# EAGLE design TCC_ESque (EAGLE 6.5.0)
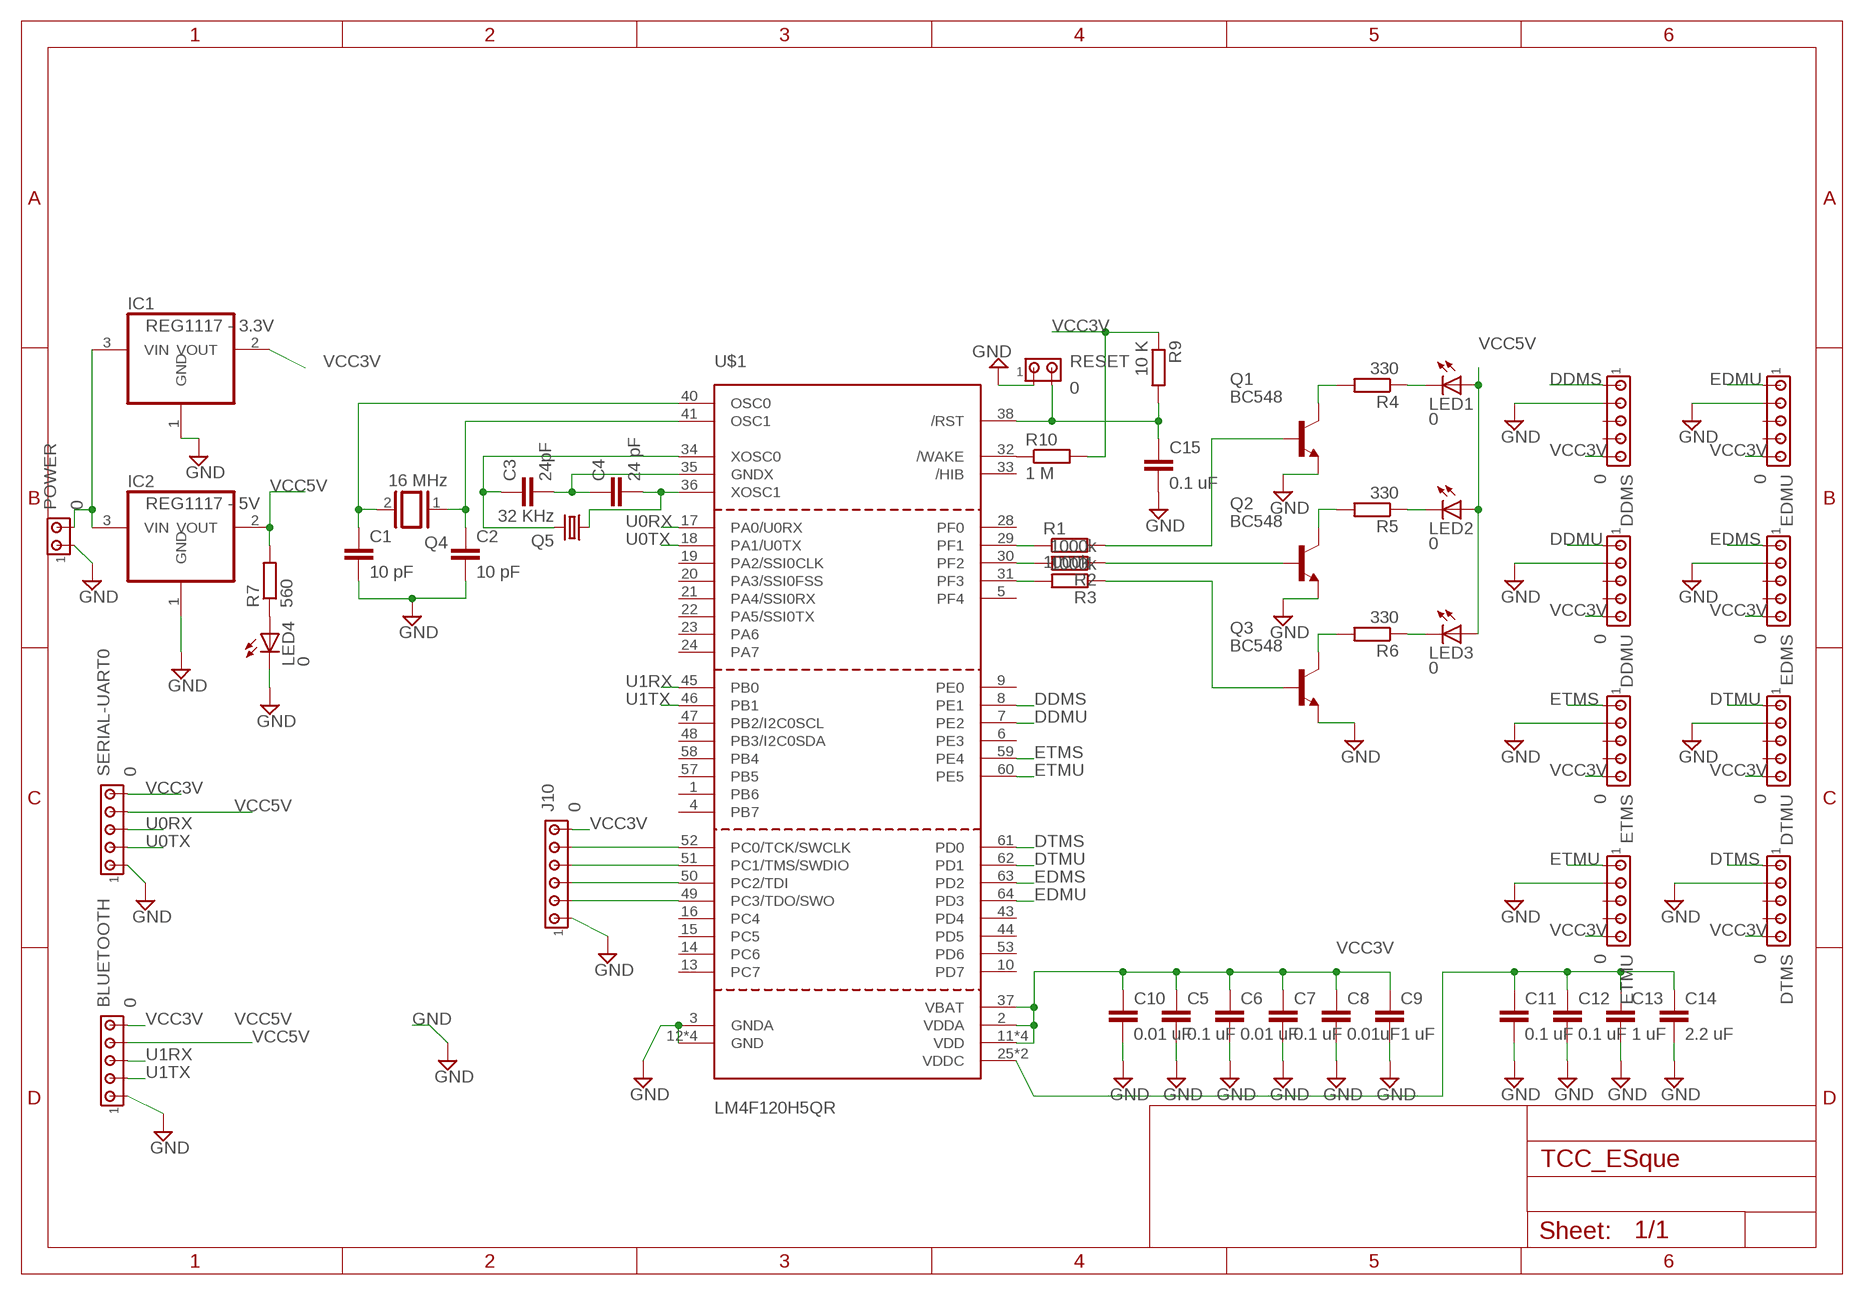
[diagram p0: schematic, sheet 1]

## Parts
BLUETOOTH  0  MTA05-100  [10X05MTA]
C1  10 pF  C2.5/6  [C2.5-6]
C2  10 pF  C2.5/6  [C2.5-6]
C3  24pF  C2.5/6  [C2.5-6]
C4  24 pF  C2.5/6  [C2.5-6]
C5  0.1 uF  C2.5/6  [C2.5-6]
C6  0.01 uF  C2.5/6  [C2.5-6]
C7  0.1 uF  C2.5/6  [C2.5-6]
C8  0.01uF  C2.5/6  [C2.5-6]
C9  1 uF  C2.5/6  [C2.5-6]
C10  0.01 uF  C2.5/6  [C2.5-6]
C11  0.1 uF  C2.5/6  [C2.5-6]
C12  0.1 uF  C2.5/6  [C2.5-6]
C13  1 uF  C2.5/6  [C2.5-6]
C14  2.2 uF  C2.5/6  [C2.5-6]
C15  0.1 uF  C2.5/6  [C2.5-6]
DDMS  0  MTA05-100  [10X05MTA]
DDMU  0  MTA05-100  [10X05MTA]
DTMS  0  MTA05-100  [10X05MTA]
DTMU  0  MTA05-100  [10X05MTA]
EDMS  0  MTA05-100  [10X05MTA]
EDMU  0  MTA05-100  [10X05MTA]
ETMS  0  MTA05-100  [10X05MTA]
ETMU  0  MTA05-100  [10X05MTA]
IC1  REG1117 - 3.3V  REG1117  [SOT223]
IC2  REG1117 - 5V  REG1117  [SOT223]
J10  0  MTA06-100  [10X06MTA]
LED1  0  LED5MM  [LED5MM]
LED2  0  LED5MM  [LED5MM]
LED3  0  LED5MM  [LED5MM]
LED4  0  LED5MM  [LED5MM]
POWER  0  MTA02-156  [1X2MTA]
Q1  BC548  [TO92-EBC]
Q2  BC548  [TO92-EBC]
Q3  BC548  [TO92-EBC]
Q4  16 MHz  XTAL/S  [QS]
Q5  32 KHz  CRYSTALTC26H  [TC26H]
R1  1000k  R-EU_0204/7  [0204/7]
R2  1000k  R-EU_0204/7  [0204/7]
R3  1000k  R-EU_0204/7  [0204/7]
R4  330  R-EU_0204/7  [0204/7]
R5  330  R-EU_0204/7  [0204/7]
R6  330  R-EU_0204/7  [0204/7]
R7  560  R-EU_0204/7  [0204/7]
R9  10 K  R-EU_0204/7  [0204/7]
R10  1 M  R-EU_0204/7  [0204/7]
RESET  0  MTA02-156  [1X2MTA]
SERIAL-UART0  0  MTA05-100  [10X05MTA]
U$1  LM4F120H5QR  [LQFP64]

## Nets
DDMS: DDMS.1 U$1.8(PE1)
DDMU: DDMU.1 U$1.7(PE2)
DTMS: DTMS.1 U$1.61(PD0)
DTMU: DTMU.1 U$1.62(PD1)
EDMS: EDMS.1 U$1.63(PD2)
EDMU: EDMU.1 U$1.64(PD3)
ETMS: ETMS.1 U$1.59(PE4)
ETMU: ETMU.1 U$1.60(PE5)
GND: BLUETOOTH.1 C1.2 C2.2 C5.2 C6.2 C7.2 C8.2 C9.2 C10.2 C11.2 C12.2 C13.2 C14.2 C15.2 DDMS.2 DDMU.2 DTMS.2 DTMU.2 EDMS.2 EDMU.2 ETMS.2 ETMU.2 IC1.1(GND) IC2.1(GND) J10.6 LED4.K(C) POWER.1 Q1.E Q2.E Q3.E RESET.1 SERIAL-UART0.1 U$1.3(GNDA) U$1.12(GND) U$1.27(GND) U$1.39(GND) U$1.55(GND)
JTAG: J10.2 U$1.52(PC0/TCK/SWCLK)
N$1: R1.1 U$1.29(PF1)
N$2: R2.2 U$1.30(PF2)
N$3: R3.2 U$1.31(PF3)
N$4: Q1.B R1.2
N$5: C1.1 Q4.2 U$1.40(OSC0)
N$6: J10.5 U$1.49(PC3/TDO/SWO)
N$7: C3.1 Q5.2 U$1.34(XOSC0)
N$8: C4.2 Q5.1 U$1.36(XOSC1)
N$9: Q2.B R2.1
N$10: Q3.B R3.1
N$11: C3.2 C4.1 U$1.35(GNDX)
N$12: Q1.C R4.2
N$13: LED1.K(C) R4.1
N$14: LED4.A R7.1
N$15: J10.4 U$1.50(PC2/TDI)
N$16: Q2.C R5.2
N$17: Q3.C R6.2
N$18: LED3.K(C) R6.1
N$19: LED2.K(C) R5.1
N$20: J10.3 U$1.51(PC1/TMS/SWDIO)
N$21: R10.1 U$1.32(/WAKE)
N$22: C15.1 R9.2 RESET.2 U$1.38(/RST)
N$23: IC1.3(VIN) IC2.3(VIN) POWER.2
N$24: C11.1 C12.1 C13.1 C14.1 U$1.25(VDDC) U$1.56(VDDC)
N$25: C2.1 Q4.1 U$1.41(OSC1)
U0RX: SERIAL-UART0.3 U$1.17(PA0/U0RX)
U0TX: SERIAL-UART0.2 U$1.18(PA1/U0TX)
U1RX: BLUETOOTH.3 U$1.45(PB0)
U1TX: BLUETOOTH.2 U$1.46(PB1)
VCC3V: BLUETOOTH.5 C5.1 C6.1 C7.1 C8.1 C9.1 C10.1 DDMS.5 DDMU.5 DTMS.5 DTMU.5 EDMS.5 EDMU.5 ETMS.5 ETMU.5 IC1.2(VOUT) J10.1 R9.1 R10.2 SERIAL-UART0.5 U$1.2(VDDA) U$1.11(VDD) U$1.26(VDD) U$1.37(VBAT) U$1.42(VDD) U$1.54(VDD)
VCC5V: BLUETOOTH.4 IC2.2(VOUT) LED1.A LED2.A LED3.A R7.2 SERIAL-UART0.4
Unconnected: DDMS.3 DDMS.4 DDMU.3 DDMU.4 DTMS.3 DTMS.4 DTMU.3 DTMU.4 EDMS.3 EDMS.4 EDMU.3 EDMU.4 ETMS.3 ETMS.4 ETMU.3 ETMU.4 U$1.1(PB6) U$1.4(PB7) U$1.5(PF4) U$1.6(PE3) U$1.9(PE0) U$1.10(PD7) U$1.13(PC7) U$1.14(PC6) U$1.15(PC5) U$1.16(PC4) U$1.19(PA2/SSI0CLK) U$1.20(PA3/SSI0FSS) U$1.21(PA4/SSI0RX) U$1.22(PA5/SSI0TX) U$1.23(PA6) U$1.24(PA7) U$1.28(PF0) U$1.33(/HIB) U$1.43(PD4) U$1.44(PD5) U$1.47(PB2/I2C0SCL) U$1.48(PB3/I2C0SDA) U$1.53(PD6) U$1.57(PB5) U$1.58(PB4)

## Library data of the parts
BLUETOOTH DDMS DDMU DTMS DTMU EDMS EDMU ETMS ETMU SERIAL-UART0 = con-amp:MTA05-100: AMP connector
C1-C15 = capacitor-wima:C: CAPACITOR
IC1 IC2 = burr-brown:REG1117: 800mA and 1A Low Dropout (LDO) Positive Regulator 1.8V, 2.5V, 2.85V, 3.3V, 5V, and Adj; MPN: REG1117; OC_FARNELL: 1097566; OC_NEWARK: 14P6981
J10 = con-amp:MTA06-100: AMP connector
LED1-LED4 = led:LED: LED
POWER RESET = con-amp:MTA02-156: AMP connector
Q1-Q3 = transistor-npn:BC548*: NPN Transistor
Q4 = special:XTAL/S: CRYSTAL
Q5 = crystal:CRYSTAL: CRYSTAL; OC_FARNELL: unknown; OC_NEWARK: unknown
R1 = resistor:R-EU_: RESISTOR, European symbol
R2-R7 R9 R10 = rcl:R-EU_: RESISTOR, European symbol
U$1 = fabhack:LM4F120H5QR: LM4F120H5QR Cortex-M4F from the LM4F120 Series.

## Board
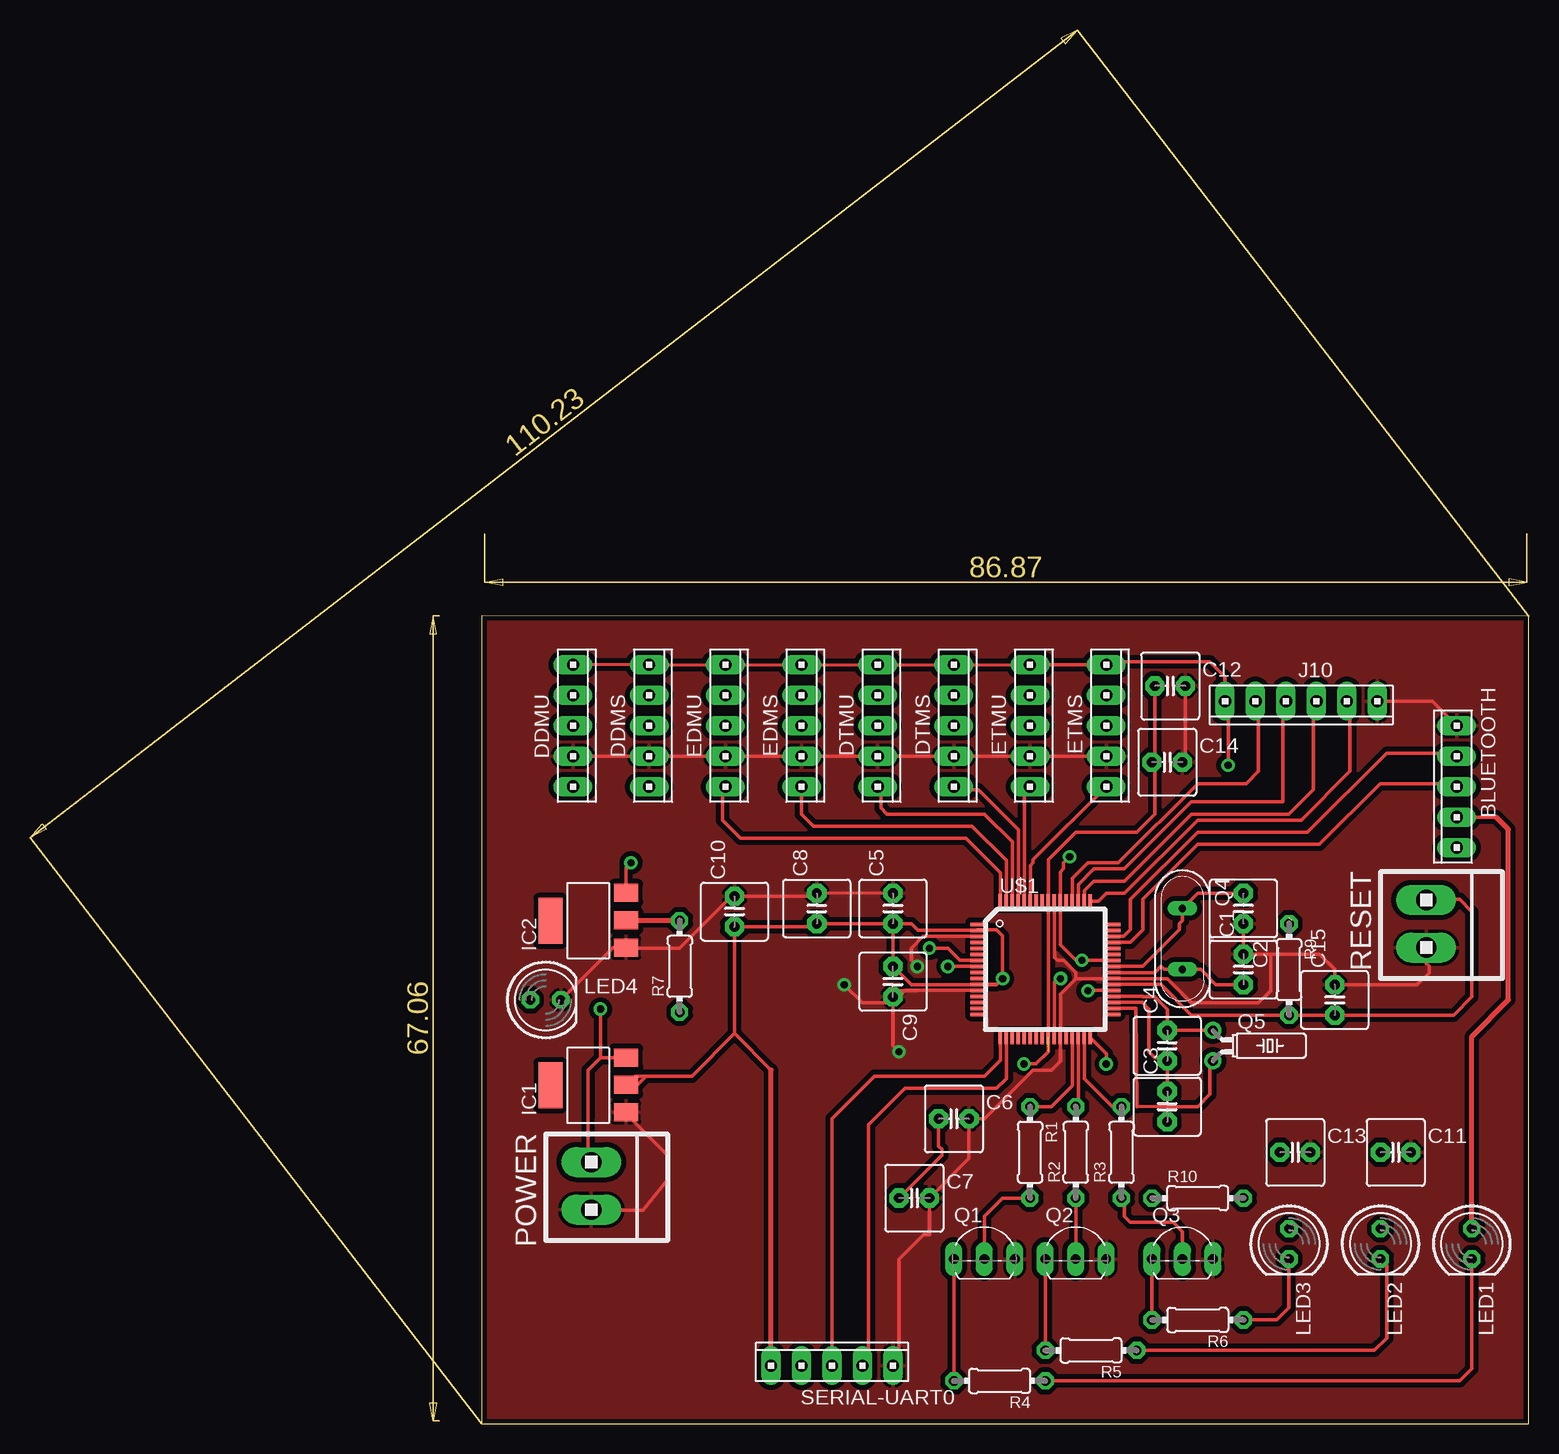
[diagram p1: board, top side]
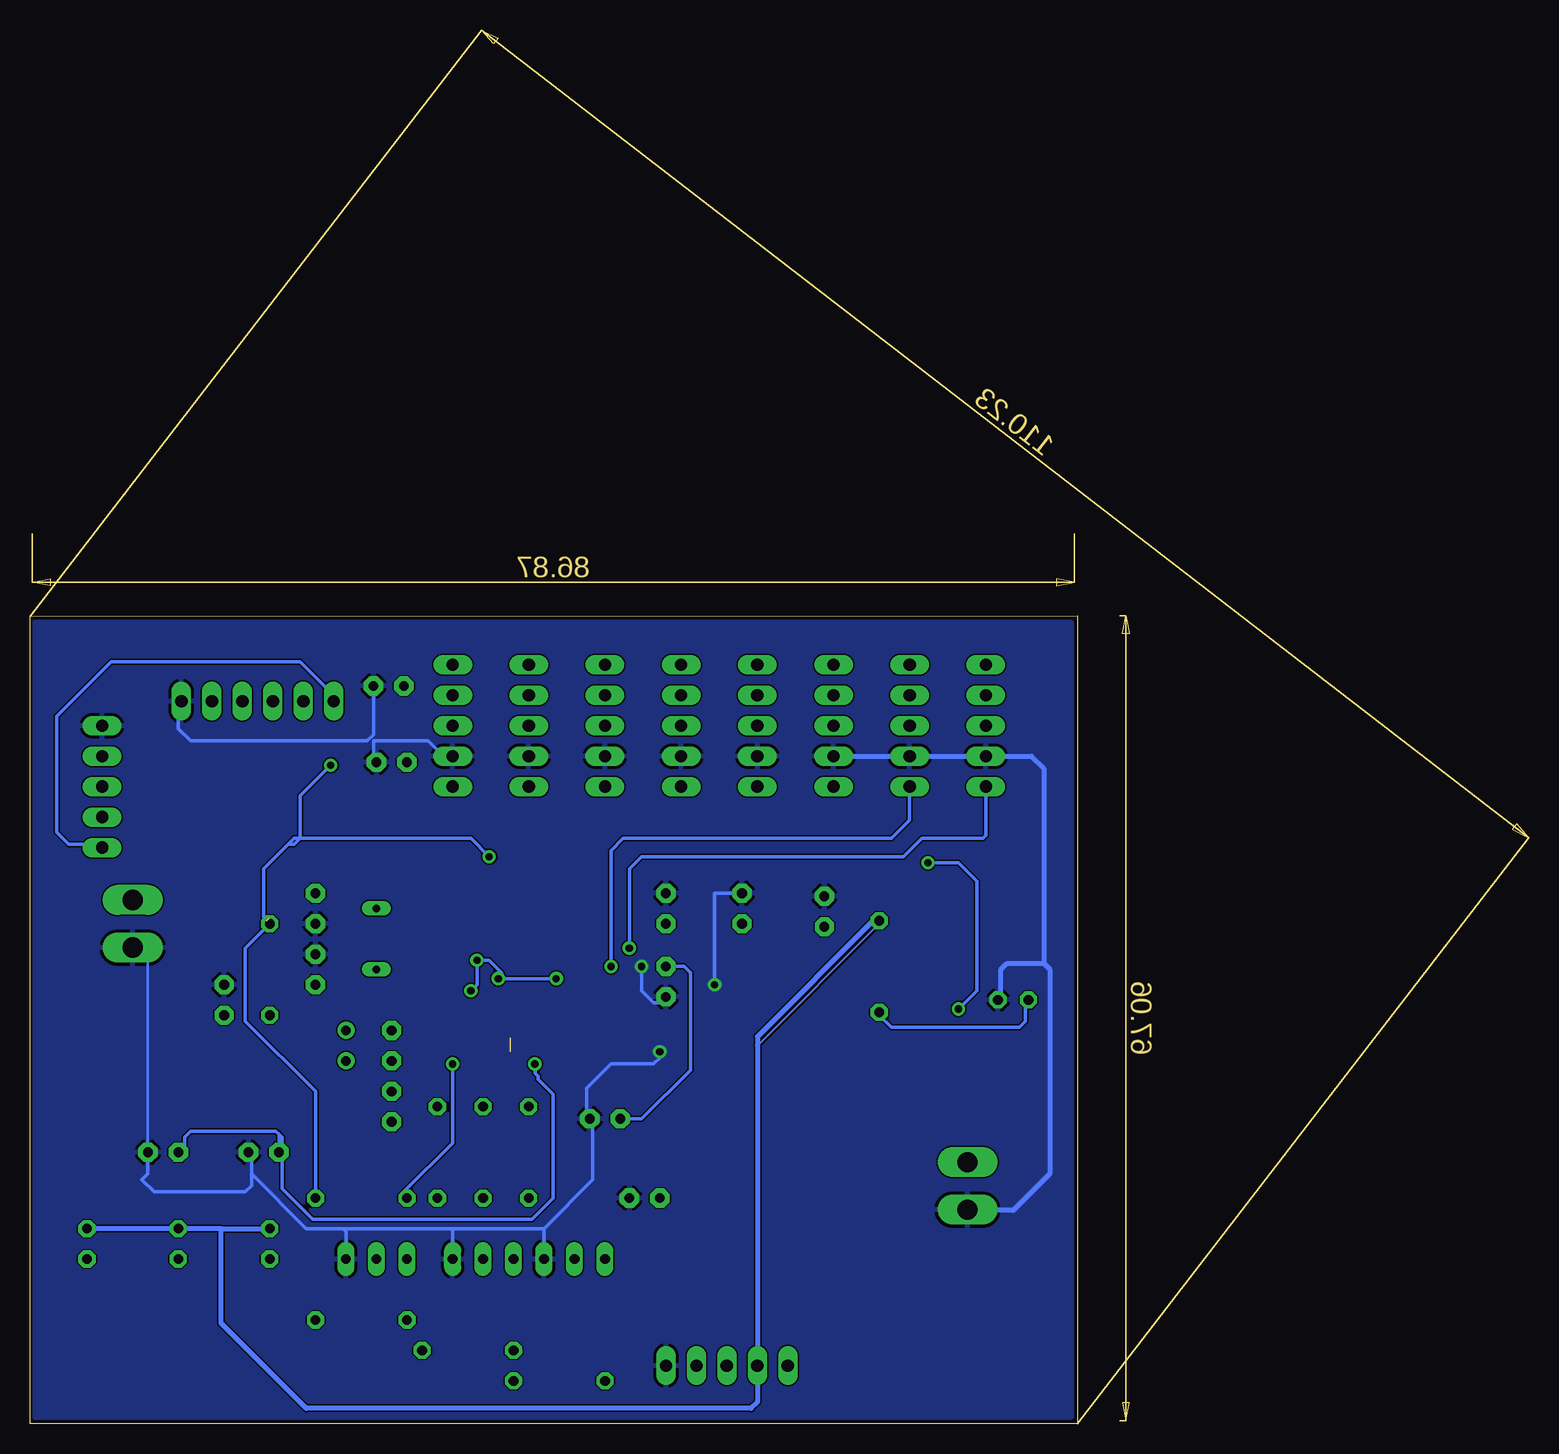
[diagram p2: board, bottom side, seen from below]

Size 124.95 x 116.13 mm. Coordinates in mm from the lower left corner, seen from the top.
Outline: 37.65,0 124.95,0 124.95,67.3 37.64,67.31 37.65,0
Copper layers (1*16): Top 0.035mm / dielectric 1.5mm / Bottom 0.035mm
Design rules "SparkFun *": minimum track width 8mil, minimum drill 23mil, track to track 5mil, track to pad 5mil, pad to pad 5mil, via to via 5mil, smd to smd 5mil, copper to edge 5mil, drill to drill 5mil, minimum pad ring 12mil, minimum via ring 10mil, stop-mask expansion 4mil, vias tented up to drill 20mil, thermal gap 10mil

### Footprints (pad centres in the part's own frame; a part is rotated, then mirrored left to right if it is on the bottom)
10X05MTA = drill 1.016 long: 1 5.08,0; 2 2.54,0; 3 0,0; 4 -2.54,0; 5 -5.08,0
C2.5-6 = drill 0.813 pad 1.6 octagon: 1 -1.27,0; 2 1.27,0
SOT223 = smd 1.499 x 2.007: 1 -2.261,-3.15; 2 0.025,-3.15; 3 2.311,-3.15 | smd 3.81 x 2.007: 4 0,3.15
10X06MTA = drill 1.016 long: 1 6.35,0; 2 3.81,0; 3 1.27,0; 4 -1.27,0; 5 -3.81,0; 6 -6.35,0
LED5MM = drill 0.813 octagon: A -1.27,0; K 1.27,0
1X2MTA = drill 1.676 long: 1 1.981,0; 2 -1.981,0
TO92-EBC = drill 0.813 long: B 0,-1.27; C -2.54,-1.27; E 2.54,-1.27
QS = drill 0.61 long: 1 -2.54,0; 2 2.54,0
TC26H = drill 0.813: 1 -1.27,0; 2 1.27,0
0204/7 = drill 0.813 octagon: 1 -3.81,0; 2 3.81,0
LQFP64 = smd 1.1 x 0.285: 1 -5.7,3.75; 2 -5.7,3.25; 3 -5.7,2.75; 4 -5.7,2.25; 5 -5.7,1.75; 6 -5.7,1.25; 7 -5.7,0.75; 8 -5.7,0.25; 9 -5.7,-0.25; 10 -5.7,-0.75; 11 -5.7,-1.25; 12 -5.7,-1.75; 13 -5.7,-2.25; 14 -5.7,-2.75; 15 -5.7,-3.25; 16 -5.7,-3.75; 33 5.7,-3.75; 34 5.7,-3.25; 35 5.7,-2.75; 36 5.7,-2.25; 37 5.7,-1.75; 38 5.7,-1.25; 39 5.7,-0.75; 40 5.7,-0.25; 41 5.7,0.25; 42 5.7,0.75; 43 5.7,1.25; 44 5.7,1.75; 45 5.7,2.25; 46 5.7,2.75; 47 5.7,3.25; 48 5.7,3.75 | smd 0.285 x 1.1: 17 -3.75,-5.7; 18 -3.25,-5.7; 19 -2.75,-5.7; 20 -2.25,-5.7; 21 -1.75,-5.7; 22 -1.25,-5.7; 23 -0.75,-5.7; 24 -0.25,-5.7; 25 0.25,-5.7; 26 0.75,-5.7; 27 1.25,-5.7; 28 1.75,-5.7; 29 2.25,-5.7; 30 2.75,-5.7; 31 3.25,-5.7; 32 3.75,-5.7; 49 3.75,5.7; 50 3.25,5.7; 51 2.75,5.7; 52 2.25,5.7; 53 1.75,5.7; 54 1.25,5.7; 55 0.75,5.7; 56 0.25,5.7; 57 -0.25,5.7; 58 -0.75,5.7; 59 -1.25,5.7; 60 -1.75,5.7; 61 -2.25,5.7; 62 -2.75,5.7; 63 -3.25,5.7; 64 -3.75,5.7

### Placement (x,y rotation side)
BLUETOOTH  118.93,53.09 90 top
C1  101.15,37.85 90 top
C2  101.15,42.93 270 top
C3  94.8,26.42 90 top
C4  94.8,31.5 90 top
C5  71.94,42.93 90 top
C6  77.02,25.4 0 top
C7  73.71,18.8 0 top
C8  65.59,42.93 90 top
C9  71.94,36.83 270 top
C10  58.73,42.67 90 top
C11  113.85,22.61 0 top
C12  95.05,61.47 0 top
C13  105.46,22.61 0 top
C14  94.8,55.12 0 top
C15  108.77,35.31 90 top
DDMS  51.62,58.17 270 top
DDMU  45.27,58.17 270 top
DTMS  77.02,58.17 270 top
DTMU  70.67,58.17 270 top
EDMS  64.32,58.17 270 top
EDMU  57.97,58.17 270 top
ETMS  89.72,58.17 270 top
ETMU  83.37,58.17 270 top
IC1  46.54,28.19 90 top
IC2  46.54,41.91 90 top
J10  105.97,60.2 180 top
LED1  120.2,14.99 270 top
LED2  112.58,14.99 270 top
LED3  104.96,14.99 270 top
LED4  42.98,35.31 0 top
POWER  46.79,19.81 270 top
Q1  79.56,14.99 0 top
Q2  87.18,14.99 0 top
Q3  96.07,14.99 0 top
Q4  96.07,40.39 270 top
Q5  98.61,31.5 270 top
R1  83.37,22.61 270 top
R2  87.18,22.61 90 top
R3  90.99,22.61 90 top
R4  80.83,3.56 180 top
R5  88.45,6.1 180 top
R6  97.34,8.64 180 top
R7  54.16,38.1 90 top
R9  104.96,37.85 270 top
R10  97.34,18.8 0 top
RESET  116.39,41.66 270 top
SERIAL-UART0  66.86,4.83 0 top
U$1  84.64,37.85 0 top

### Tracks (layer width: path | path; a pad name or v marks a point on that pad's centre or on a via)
DDMS  (via drill 0.6)
  Top 0.305: U$1.8 v76.51,38.1
  Bottom 0.305: v76.51,38.1 76.51,47.75 75.49,48.77 53.14,48.77 51.62,50.29 DDMS.1
DDMU  (via drill 0.6)
  Top 0.305: v74.98,39.62 76.51,39.62 77.52,38.61 78.92,38.61 U$1.7
  Bottom 0.305: DDMU.1 45.27,49.02 45.52,48.77 50.6,48.77 52.12,47.24 73.97,47.24 74.98,46.23 v74.98,39.62
DTMS
  Top 0.305: U$1.61 82.39,49.49 79.05,52.83 77.27,52.83 DTMS.1
DTMU
  Top 0.305: U$1.62 81.89,48.47 79.56,50.8 71.43,50.8 70.92,51.31 70.92,52.83 DTMU.1
EDMS
  Top 0.305: U$1.63 81.39,46.94 78.54,49.78 65.33,49.78 64.32,50.8 EDMS.1
EDMU
  Top 0.305: U$1.64 80.89,45.91 78.03,48.77 59.24,48.77 57.71,50.29 57.71,52.83 EDMU.1
ETMS
  Top 0.305: U$1.59 83.39,46.5 83.62,46.74 83.62,46.99 ETMS.1
ETMU
  Top 0.305: U$1.60 82.89,52.61 ETMU.1
GND  (via drill 0.6)
  Top 0.203: 50.35,25.15 50.35,26.42 IC1.1
  Top 0.254: C5.2 C8.2
  Top 0.305: C2.2 C1.2 103.43,39.12 | 103.43,39.12 107.5,39.12 108.77,37.85 C15.2 115.62,36.58 116.64,37.59 116.64,38.1 116.39,38.35 RESET.1 | 90.35,37.08 94.8,37.08 96.83,35.05 102.42,35.05 103.43,36.07 103.43,39.12 | 89.72,14.22 Q2.E | SERIAL-UART0.1 72.44,5.33 72.44,13.72 74.48,15.75 74.98,15.75 C7.2 78.29,22.1 C6.2 79.56,25.4 83.62,29.46 85.14,29.46 85.89,30.21 U$1.27 85.89,35.79 87.18,37.08 | 50.07,25.93 50.09,25.91 50.09,25.4 50.35,25.15 53.14,22.35 53.14,20.32 51.11,17.78 47.35,17.78 POWER.1 45.47,17.83 | C10.2 58.47,44.2 | LED4.K 48.59,39.65 IC2.1 49.71,39.62 54.16,39.62 58.47,43.94 C10.2 | C10.2 65.33,43.94 C8.2 | DDMU.2 DDMS.2 EDMU.2 EDMS.2 DTMU.2 DTMS.2 ETMU.2 ETMS.2 | C12.2 96.32,55.37 C14.2 | J10.6 116.89,60.2 BLUETOOTH.1 | v67.87,36.58 69.4,35.05 71.43,35.05 C9.2 72.44,36.07 73.97,36.07 74,36.1 U$1.12 72.98,36.1 71.94,35.05 71.94,31.5 v72.44,30.99 | U$1.3 74.43,40.6 73.46,39.62 73.46,38.61 v73.97,38.1 | U$1.55 85.39,38.87 85.65,38.61 86.16,38.61 87.18,37.59 87.18,37.08 | 87.18,37.08 90.32,37.08 U$1.39
  Bottom 0.203: C11.2 115.12,39.12 116.39,39.12 RESET.1
  Bottom 0.305: Q1.E 82.1,16.26 | 82.1,16.26 89.72,16.26 | 89.72,16.26 98.86,16.26 | 98.86,16.26 98.61,16 Q3.E | Q2.E 89.72,16.26 | 82.1,16.26 78.03,20.32 78.03,24.64 78.29,24.89 C6.2 78.54,25.65 78.54,27.94 76.51,29.97 72.95,29.97 72.44,30.48 v72.44,30.99 | ETMS.2 90.48,55.63 91.75,56.9 96.32,56.9 96.32,55.37 C14.2 | C12.2 96.32,57.4 96.83,56.9 111.56,56.9 112.58,57.91 112.58,59.94 J10.6 | 98.86,16.26 101.91,16.26 106.48,20.83 | 106.48,20.83 106.48,22.35 C13.2 | C11.2 115.12,20.83 115.62,20.32 114.61,19.3 106.99,19.3 106.48,19.81 106.48,20.83 | v67.87,36.58 67.87,44.2 C8.2 | v73.97,38.1 73.97,36.07 72.95,35.05 72.44,35.05 C9.2
  Bottom 0.406: LED4.K 44,35.31 44,37.85 43.49,38.35 40.44,38.35 | 40.44,38.35 39.93,37.85 39.93,20.83 42.98,17.78 46.74,17.78 POWER.1 | EDMU.2 41.46,55.63 40.44,54.61 40.44,38.35
  pour Top (isolate 0.406): 38.15,0.51 124.51,0.51 124.51,66.8 38.15,67.06
  pour Bottom: 38.41,66.8 38.15,66.8 38.15,0.51 124.51,0.51 124.51,66.8 38.15,66.8 38.15,66.55 38.41,66.8 38.15,66.8 38.15,66.29
JTAG
  Top 0.305: U$1.52 86.89,45.43 88.19,46.74 90.73,46.74 97.34,53.34 101.4,53.34 102.42,54.36 102.42,59.94 J10.2
N$1
  Top 0.305: U$1.29 86.89,28.16 85.14,26.42 R1.1
N$2
  Top 0.305: U$1.30 87.39,26.63 R2.2
N$3
  Top 0.305: U$1.31 87.89,28.75 90.22,26.42 R3.2
N$4
  Top 0.305: R1.2 81.08,18.8 79.56,17.27 Q1.B
N$5
  Top 0.305: C1.1 98.86,36.58 97.59,37.85 Q4.2 94.54,37.85 94.29,38.1 93.78,37.59 U$1.40
N$6
  Top 0.305: U$1.49 89.07,43.55 89.72,44.2 91.24,44.2 97.34,50.29 105.97,50.29 110.04,54.36 110.04,59.94 J10.5
N$7
  Top 0.254: C3.1 94.8,26.42 92.26,26.42 92.25,26.42
  Top 0.305: U$1.34 92.2,34.6 92.25,26.42 | 94.8,26.42 97.34,26.42 98.35,27.43 98.35,29.97 Q5.2
N$8
  Top 0.305: Q5.1 C4.2 94.8,34.54 93.78,35.56 92.76,35.56 92.73,35.6 U$1.36
N$9
  Top 0.305: R2.1 Q2.B
N$10
  Top 0.305: R3.1 91.24,18.54 91.24,17.27 91.75,16.76 95.3,16.76 96.07,16 Q3.B
N$11
  Top 0.305: C3.2 C4.1 94.54,30.48 93.78,30.48 93.27,30.99 93.27,34.54 92.72,35.1 U$1.35
N$12
  Top 0.305: Q1.C R4.2
N$13
  Top 0.305: R4.1 119.18,3.56 120.2,4.57 LED1.K
N$14
  Bottom 0.305: LED4.A 41.96,35.05 41.96,33.53 42.47,33.02 53.14,33.02 54.16,34.04 R7.1
N$15
  Top 0.305: U$1.50 87.89,44.4 88.7,45.21 91.24,45.21 96.83,50.8 104.96,50.8 106.99,52.83 106.99,59.94 J10.4
N$16
  Top 0.305: Q2.C R5.2
N$17
  Top 0.305: R6.2 Q3.C
N$18
  Top 0.305: R6.1 103.94,8.64 104.96,9.65 LED3.K
N$19
  Top 0.305: R5.1 112.07,6.1 113.08,7.11 113.08,13.21 LED2.K
N$20
  Top 0.305: U$1.51 87.39,44.91 88.7,46.23 91.24,46.23 96.83,51.82 104.45,51.82 104.45,59.94 J10.3
N$21  (via drill 0.6)
  Top 0.305: U$1.32 89.72,30.82 v89.72,29.97
  Bottom 0.305: v89.72,29.97 89.72,23.37 93.78,19.3 93.53,19.05 R10.1
N$22
  Top 0.305: U$1.38 94.27,36.6 96.83,34.04 R9.2 C15.1 118.67,34.04 120.2,35.56 120.2,42.67 119.18,43.69 116.44,43.69 RESET.2
N$23  (via drill 0.6)
  Top 0.305: POWER.2 46.54,22.05 46.54,29.46 47.55,30.48 | 47.55,30.48 47.58,30.51 IC1.3 49.66,30.48 47.55,30.48 | 47.55,30.48 v47.55,34.54 | v50.09,46.74 49.69,46.33 IC2.3
  Bottom 0.305: v47.55,34.54 46.03,36.07 46.03,45.21 47.55,46.74 v50.09,46.74
N$24  (via drill 0.6)  (1 unrouted)
  Top 0.305: C12.1 93.78,55.37 C14.1 93.78,54.86 93.78,50.8 92.26,49.28 87.18,49.28 84.89,46.99 U$1.56 84.89,30.99 83.87,29.97 v82.86,29.97
  Bottom 0.305: C13.1 104.19,24.13 | 104.19,24.13 104.45,24.38 111.56,24.38 112.07,23.88 112.07,23.11 C11.1 | 104.19,24.13 103.94,23.88 103.94,19.56 101.4,17.02 83.11,17.02 81.33,18.8 81.33,27.43 82.6,28.7 82.6,28.96 82.86,29.21 v82.86,29.97
N$25
  Top 0.305: U$1.41 92.76,38.1 95.81,41.15 95.81,41.66 96.07,41.91 Q4.1 97.34,44.2 C2.1
U0RX
  Top 0.305: SERIAL-UART0.3 66.86,25.4 70.41,28.96 79.56,28.96 80.89,30.29 U$1.17
U0TX
  Top 0.305: SERIAL-UART0.2 69.9,5.33 69.9,24.89 72.95,27.94 80.57,27.94 81.39,28.75 U$1.18
U1RX
  Top 0.305: U$1.45 91.71,40.1 92.76,41.15 92.76,43.69 97.34,48.26 107.5,48.26 112.58,53.34 118.67,53.34 BLUETOOTH.3
U1TX
  Top 0.305: U$1.46 91.2,40.6 91.75,41.15 91.75,43.69 97.34,49.28 106.48,49.28 113.08,55.88 118.67,55.88 BLUETOOTH.2
VCC3V  (via drill 0.6)  (1 unrouted)
  Top 0.254: DDMU.5 DDMS.5 EDMU.5 EDMS.5 DTMU.5 DTMS.5 ETMU.5
  Top 0.305: C7.1 76,22.35 76,22.86 75.75,23.11 C6.1 | 50.42,28.96 51.36,28.96 | 51.36,28.96 55.17,28.96 58.73,32.51 | 58.73,32.51 C10.1 65.33,41.4 C8.1 C5.1 | C5.1 73.46,41.66 74.02,41.1 U$1.2 78.99,41.15 80.57,41.15 81.08,40.64 v81.08,37.08 80.57,36.58 | C5.1 C9.1 73.46,36.58 80.57,36.58 | U$1.11 80.55,36.6 80.57,36.58 | 61.78,29.46 58.73,32.51 | ETMU.5 ETMS.5 89.97,63.5 98.35,63.5 99.62,62.23 J10.1 99.88,59.94 v99.88,54.86 | 119.18,47.75 BLUETOOTH.5 | v86.67,47.24 86.16,46.74 86.16,46.23 85.89,45.95 U$1.54 85.89,39.9 87.18,38.61 v87.68,38.61 v87.7,38.6 U$1.42 | U$1.26 85.39,36.82 v85.91,37.08 | U$1.37 88.22,36.1 v88.19,36.07 | R9.1 105.21,41.91 | IC1.2 50.63,28.22 51.36,28.96
  Top 0.406: SERIAL-UART0.5 61.78,29.46
  Bottom 0.305: J10.1 99.62,60.71 102.42,63.5 118.16,63.5 122.74,58.93 122.74,49.28 121.72,48.26 119.18,48.26 BLUETOOTH.5 | v86.67,47.24 88.19,48.77 102.42,48.77 | 102.42,48.77 102.92,48.26 103.43,48.26 | 104.96,42.16 105.46,41.66 | 102.42,48.77 102.92,48.77 105.46,46.23 105.46,42.16 R9.1 106.99,39.62 106.99,33.53 101.15,27.69 R10.2 | 102.42,48.77 102.42,52.32 v99.88,54.86 | C6.1 73.97,25.4 69.9,29.46 69.9,37.59 70.41,38.1 C9.1 | v88.19,36.07 87.68,36.58 v87.68,38.61 86.67,38.61 85.65,37.59 v85.91,37.08 v81.08,37.08
VCC5V
  Top 0.305: 122.23,50.55 BLUETOOTH.4
  Top 0.406: IC2.2 54.13,41.93 R7.2 | LED1.A 120.2,32.26 123.24,35.31 123.24,49.53 122.23,50.55
  Bottom 0.203: 64.32,31.5 54.16,41.66 R7.2
  Bottom 0.406: 54.66,41.91 64.32,32.26 64.32,31.5 SERIAL-UART0.4 64.32,1.78 64.82,1.27 101.91,1.27 109.02,8.38 109.02,16.26 | 109.02,16.26 LED2.A LED1.A | 109.02,16.26 LED3.A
